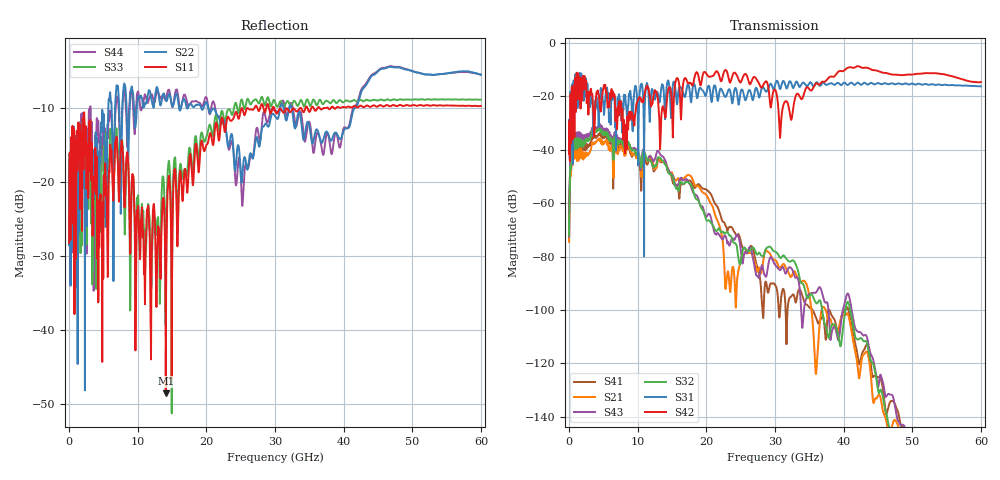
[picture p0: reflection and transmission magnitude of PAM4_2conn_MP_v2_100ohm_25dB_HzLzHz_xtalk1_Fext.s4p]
! Info: Touchstone file created by Circ.  Input file=FAB50GbE_2conn_Midplane_Examax_Topo2_v2_100ohm_25dB_HzLzHz.circ
# Hz S RI R 50
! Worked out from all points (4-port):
!   6000 points, 10 MHz to 60 GHz, reference 50 ohm
!   strongest paths, dB at 10 MHz, 15.01 GHz, 30.01 GHz, 45.01 GHz, 60 GHz:
!     S42: -41.6, -24.7, -17.5, -10.5, -14.7
!     S31: -41.2, -18.9, -15.8, -15.0, -16.3
!     S32: -72.1, -49.8, -78.1, -130.0, -170.7
!     S43: -72.5, -49.5, -83.1, -128.8, -171.2
!     S21: -74.5, -48.6, -81.3, -132.1, -164.9
!     S41: -69.7, -50.9, -90.6, -125.1, -168.8
!   lowest |S11| = -48.6 dB at 14.09 GHz (marker M1), VSWR 1.01, Z = 50.3 - j0.131 ohm
!   |S11| at or under -10 dB: start of sweep to 27.01 GHz; 29.87 GHz to 34.45 GHz (4.581 GHz wide, 14.2 % of centre); 36.49 GHz to 37.52 GHz (1.034 GHz wide, 2.79 % of centre)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
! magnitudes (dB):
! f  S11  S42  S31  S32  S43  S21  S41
! 10 MHz  -28.3  -41.6  -41.2  -72.1  -72.5  -74.5  -69.7
! 630 MHz  -16.6  -16.4  -14.7  -37.9  -35.5  -40.8  -36.9
! 3.59 GHz  -19.9  -28.2  -34.9  -32.6  -31.2  -37.3  -34.6
! 14.09 GHz  -48.6  -26.9  -21.9  -45.6  -44.6  -45.2  -44.7
! 22.85 GHz  -12.6  -10.2  -20.1  -71.0  -72.6  -91.4  -68.7
! 30.8 GHz  -10.2  -33.6  -17.1  -80.6  -85.1  -84.2  -98.2
! 60 GHz  -9.8  -14.7  -16.3  -170.7  -171.2  -164.9  -168.8
